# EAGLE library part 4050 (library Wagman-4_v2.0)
Hex non-inverting BUFFER
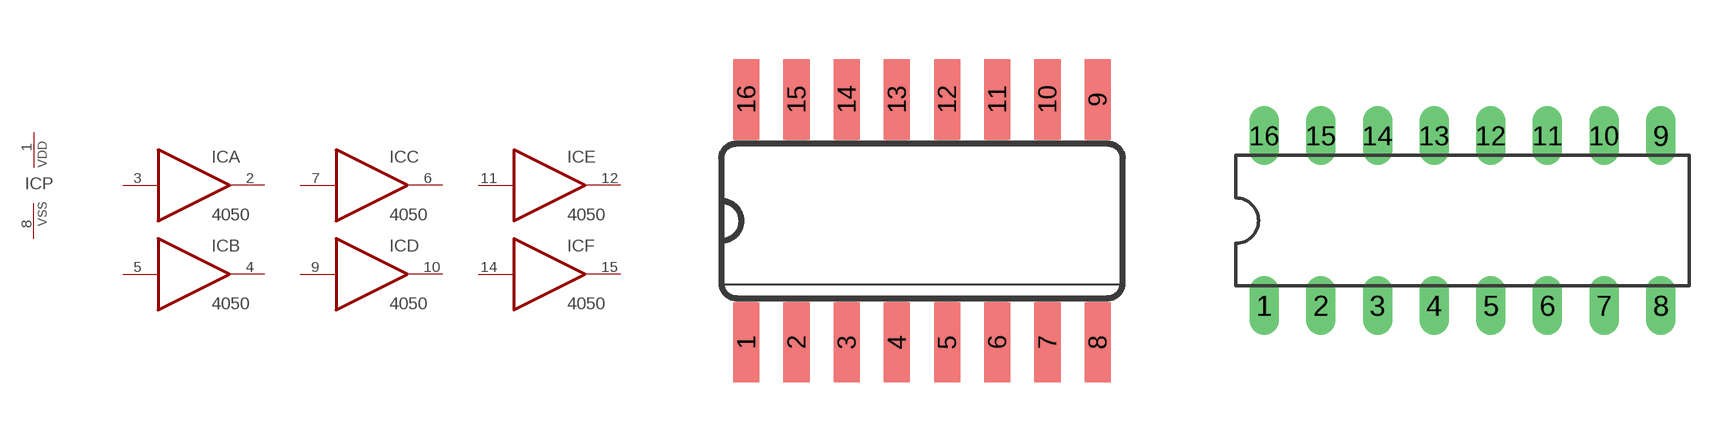
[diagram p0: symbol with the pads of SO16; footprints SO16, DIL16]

Designator prefix IC; gates A=4050 B=4050 C=4050 D=4050 E=4050 F=4050 P=PWRN

## 4050D  [SO16]
1  P:VDD  pwr
2  A:O  out
3  A:I  in
4  B:O  out
5  B:I  in
6  C:O  out
7  C:I  in
8  P:VSS  pwr
9  D:I  in
10  D:O  out
11  E:I  in
12  E:O  out
14  F:I  in
15  F:O  out

## 4050N  [DIL16]
Pads as for SO16

## Footprint SO16 (pad centres in mm)
Small Outline package 150 mil
smd 0.66 x 2.032: 1 -4.445,-3.073; 2 -3.175,-3.073; 3 -1.905,-3.073; 4 -0.635,-3.073; 5 0.635,-3.073; 6 1.905,-3.073; 7 3.175,-3.073; 8 4.445,-3.073; 9 4.445,3.073; 10 3.175,3.073; 11 1.905,3.073; 12 0.635,3.073; 13 -0.635,3.073; 14 -1.905,3.073; 15 -3.175,3.073; 16 -4.445,3.073

## Footprint DIL16 (pad centres in mm)
Dual In Line Package
drill 0.813 long: 1 -8.89,-3.81; 2 -6.35,-3.81; 3 -3.81,-3.81; 4 -1.27,-3.81; 5 1.27,-3.81; 6 3.81,-3.81; 7 6.35,-3.81; 8 8.89,-3.81; 9 8.89,3.81; 10 6.35,3.81; 11 3.81,3.81; 12 1.27,3.81; 13 -1.27,3.81; 14 -3.81,3.81; 15 -6.35,3.81; 16 -8.89,3.81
